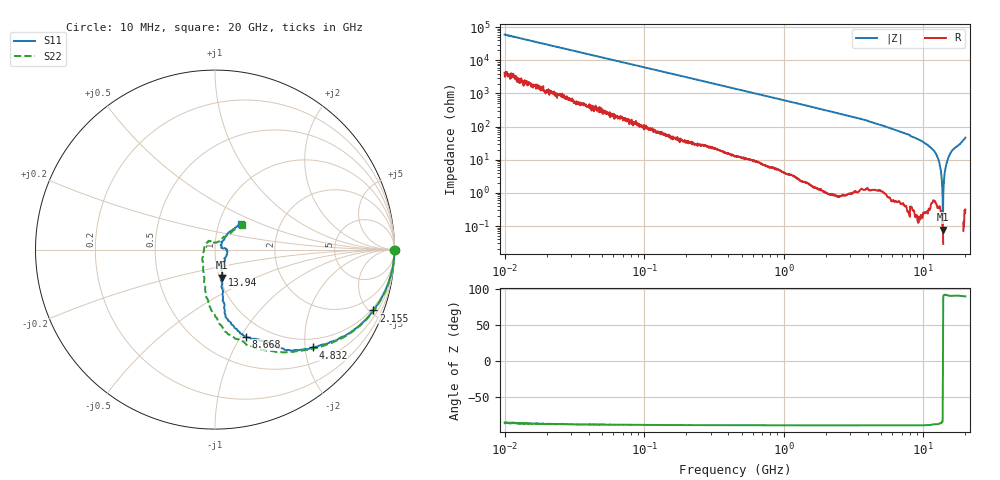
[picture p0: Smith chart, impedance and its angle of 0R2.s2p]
!Keysight Technologies,P5008B,MY61100088,A.16.20.02
!Date: Friday, August 30, 2024 10:27:07
!Correction: S11(C  2-Port  )
!S21(C  2-Port  )
!S12(C  2-Port  )
!S22(C  2-Port  )
!S2P File: Measurements: S11, S21, S12, S22:Log Frequency Sweep
# Hz S  dB  R 50
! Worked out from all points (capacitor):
!   1601 points, 10 MHz to 20 GHz, reference 50 ohm
!   read as one part in series: C = 266 fF near 10.39 MHz
!   lowest |Z| = 79 mohm at 13.81 GHz (marker M1)
!   series resonance near 13.81 GHz, so ESL is about 500 pH
!   S11 on the Smith chart (normalised r, x): 10 MHz: open; 2.155 GHz: 0.82, -5.27; 4.832 GHz: 0.81, -2.16; 8.668 GHz: 0.80, -1.05; 13.94 GHz: 1.03, -0.30; 20 GHz: 1.27, +0.38
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1e7  0.00 -0.1  -55.52 85.9  -55.47 86.4  -0.00 -0.1
3.555162e7  -0.00 -0.4  -44.67 87.9  -44.66 88.0  -0.00 -0.4
1.263918e8  -0.01 -1.3  -33.81 87.9  -33.81 87.9  -0.00 -1.3
4.472136e8  -0.03 -4.5  -22.95 84.9  -22.95 84.9  -0.03 -4.6
8.738125e8  -0.09 -8.7  -17.22 80.7  -17.23 80.7  -0.09 -9.0
1.589917e9  -0.28 -15.5  -12.22 74.0  -12.22 74.0  -0.28 -16.1
2.154843e9  -0.48 -21.0  -9.80 68.5  -9.80 68.5  -0.49 -21.6
3.432446e9  -1.16 -32.7  -6.37 56.7  -6.37 56.7  -1.16 -33.3
4.832257e9  -2.27 -45.0  -3.98 43.8  -3.99 43.7  -2.28 -46.2
5.652411e9  -2.97 -52.3  -3.08 36.7  -3.09 36.6  -2.98 -53.4
7.697294e9  -4.83 -62.5  -1.71 23.3  -1.71 23.3  -4.83 -69.8
8.667956e9  -5.76 -70.5  -1.31 16.1  -1.32 16.0  -5.79 -76.2
1.191646e10  -9.41 -80.8  -0.52 0.8  -0.52 0.7  -9.47 -93.9
1.273595e10  -11.45 -80.4  -0.29 -2.8  -0.29 -2.9  -11.60 -100.8
1.380717e10  -15.85 -75.7  -0.03 -8.6  -0.04 -8.7  -16.08 -114.1
1.393898e10  -16.58 -75.1  -0.01 -9.3  -0.01 -9.5  -16.85 -116.3
1.547463e10  -23.05 -42.8  0.05 -18.4  0.05 -18.5  -24.27 -172.9
1.653881e10  -24.14 -0.6  0.05 -23.9  0.05 -24.0  -24.93 129.9
1.776035e10  -28.84 16.3  0.06 -30.5  0.06 -30.6  -28.86 103.7
1.836088e10  -26.22 40.5  0.05 -34.0  0.04 -34.2  -26.41 67.7
1.943798e10  -17.57 50.0  -0.06 -40.8  -0.06 -41.0  -17.69 46.1
2e10  -13.82 45.1  -0.18 -44.9  -0.18 -45.1  -13.73 42.2
